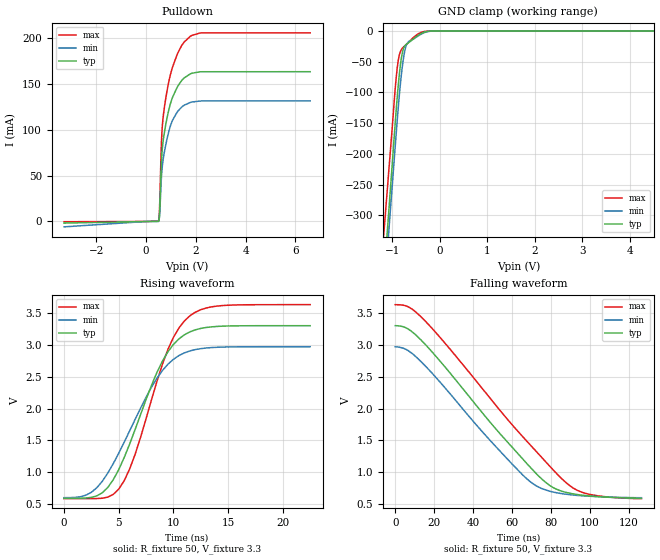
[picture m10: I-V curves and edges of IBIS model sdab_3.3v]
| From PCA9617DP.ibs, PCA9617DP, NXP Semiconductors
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[Model]   sdab_3.3v
Model_type Open_drain
Vref=3.300E+00
Rref=1.350E+03
Cref=5.000E-11
Vmeas=1.650E+00
C_comp   8.050E-13   7.840E-13   8.260E-13
[Voltage Range]   3.300E+00   2.970E+00   3.630E+00
[POWER Clamp Reference]   3.300E+00   2.970E+00   3.630E+00
[GND Clamp Reference]   0.000E+00   0.000E+00   0.000E+00
[Pullup Reference]   3.300E+00   2.970E+00   3.630E+00
[Pulldown Reference]   0.000E+00   0.000E+00   0.000E+00
[Temperature Range]   25   85   -40
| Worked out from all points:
|   slope of the pulldown table from 0 to 0.495 V, typ, clamps not added: 3.71 kohm
|   GND clamp passes 1 mA (typ) near -0.29 V on its own axis
|   rising waveform, R_fixture 50, V_fixture 3.3: 20-80 % time 3.8ns typ, 4.28ns min, 3.44ns max; typ from 0.593 V to 3.3 V
|   falling waveform, R_fixture 50, V_fixture 3.3: 20-80 % time 45.1ns typ, 41.1ns min, 50.7ns max; typ from 3.3 V to 0.593 V
[GND Clamp]
-3.3V     -2.642A    -2.605A    -2.395A
-1V       -212mA     -247.6mA   -152.7mA
-940mV    -147.9mA   -185.9mA   -92.12mA
-880mV    -90.26mA   -126.9mA   -48.79mA
-840mV    -59.92mA   -92.03mA   -34.95mA
-800mV    -38.5mA    -62.74mA   -28.77mA
-740mV    -24.36mA   -32.34mA   -24.21mA
-700mV    -21.13mA   -21.48mA   -21.25mA
-660mV    -18.99mA   -17.13mA   -18.12mA
-400mV    -4.117mA   -5.255mA   -2.294mA
-160mV    0A         0A         0A
6.6V      0A         0A         0A
[Pulldown]
-3.3V     -1.733mA   -5.84mA    -255uA
500mV     134.8uA    96.13uA    436.8uA
540mV     7.493mA    5.051mA    12.52mA
600mV     53.43mA    39.39mA    71.96mA
640mV     74.86mA    56.47mA    98.39mA
700mV     90.35mA    69.89mA    116.7mA
820mV     109.6mA    87.13mA    138.7mA
980mV     128.4mA    104.1mA    160mA
1.24V     145.6mA    118.7mA    181.2mA
1.78V     160.8mA    129.6mA    201.7mA
2.26V     163.1mA    131.3mA    205.4mA
6.6V      163.1mA    131.3mA    205.5mA
[Rising Waveform]
R_fixture = 50
V_fixture = 3.3
V_fixture_min = 2.97
V_fixture_max = 3.63
0s        593.4mV    601.8mV    586.7mV
2.5ns     606.1mV    685.9mV    586.7mV
4ns       761.6mV    987.2mV    610.5mV
5ns       1.041V     1.299V     735.5mV
6.5ns     1.672V     1.83V      1.283V
9ns       2.746V     2.598V     2.698V
10ns      3.006V     2.773V     3.117V
11.5ns    3.203V     2.904V     3.454V
14ns      3.288V     2.962V     3.608V
22.5ns    3.3V       2.97V      3.63V
[Falling Waveform]
R_fixture = 50
V_fixture = 3.3
V_fixture_min = 2.97
V_fixture_max = 3.63
0s        3.3V       2.97V      3.63V
7ns       3.241V     2.902V     3.591V
15.5ns    3.004V     2.667V     3.37V
52ns      1.67V      1.393V     2.04V
65.5ns    1.21V      958.6mV    1.559V
72ns      994.3mV    796.8mV    1.342V
81.5ns    755.2mV    688.5mV    1.027V
93.5ns    651.7mV    638.2mV    718.7mV
104.5ns   618mV      618.2mV    630.2mV
126.5ns   593.4mV    601.8mV    586.7mV
[Ramp]
dV/dt_r   1.6239E+00/3.7850E-09   1.4209E+00/4.2700E-09   1.8260E+00/3.4110E-09
dV/dt_f   1.6239E+00/4.5088E-08   1.4209E+00/4.1083E-08   1.8260E+00/5.0737E-08
R_load = 50
